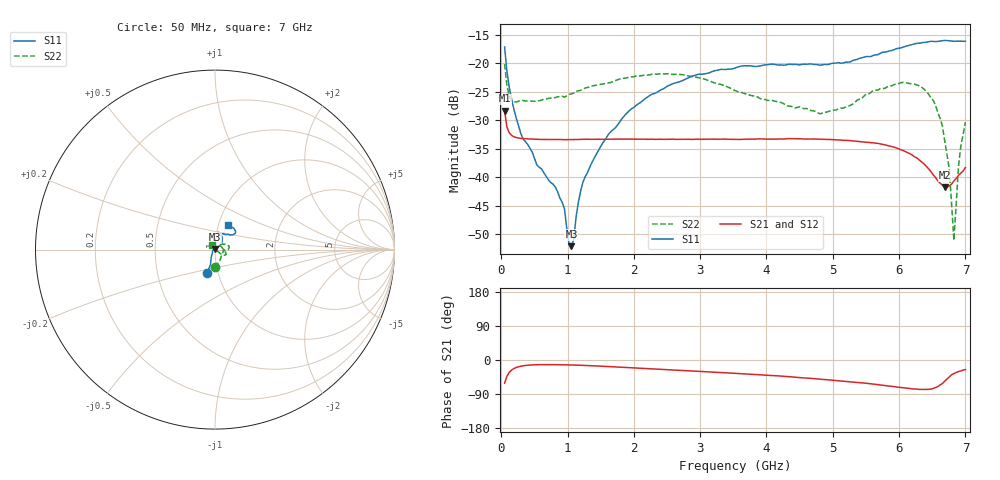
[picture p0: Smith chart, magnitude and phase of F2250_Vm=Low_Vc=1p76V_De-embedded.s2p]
! Integrated Device Technology
! Corporate Headquarters
! 6024 Silver Creek Valley Road
! San Jose, CA 95138  USA
! Phone:  1-408-284-8200
! Toll Free:  1-800-223-1366
! Webpage:  http://www.idt.com/
! Timing and RF Division
! 515 Groton Road, Suite 102
! Westford, MA 01886-6024
! Device:  F2250
! Description: Voltage Variable RF Attenuator
! Frequency:  50.0 -  6000.00 MHz
! Package:  3x3 mm Thin QFN Plastic Package: 16 pin
! Ports:  2 RF, 3 DC
!  Pin  1  = GND
!  Pin  2  = NC
!  Pin  3  = RF1  = Port 1
!  Pin  4  = NC
!  Pin  5  = GND
!  Pin  6  = GND
!  Pin  7  = GND
!  Pin  8  = GND
!  Pin  9  = NC
!  Pin 10  = RF2  = Port 2
!  Pin 11  = NC
!  Pin 12  = GND
!  Pin 13  = GND
!  Pin 14  = VCNTRL
!  Pin 15  = VDD
!  Pin 16  = VMODE
! Vcntrl:  1.760 Volts
! Vmode:  +0.000 Volts
! Vdd:  +3.30  Volts
! Current:  1.187 mA
! Data:  The device was measured on a the F2250 evaluation board which has
!  individual transmission lines to the RF pins.  Data was collected
!  using a calibrated network analyzer.  The evaluation board was
!  de-embedded using a TRL calibration technique.
!  The reference plane is the edge of the package pin.
! Misc:  SN 10
!  Action Tracker AT0258
! Date Measured:  2014-11-26
! Date:  2015-10-15  MJV
! Note:
!  Integrated Device Technology supplies this data as a sample of measured
!  data at the package pin for this product.  Your particular data for this
!  product may vary.
!  Data was taken at 25 degrees C.
!  Integrated Device Technology reserves the right to change this data at anytime.
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# GHz S dB R 50
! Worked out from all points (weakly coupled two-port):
!   201 points, 50 MHz to 7 GHz, reference 50 ohm
!   highest |S21| = -28.35 dB at 50 MHz (marker M1); lowest = -41.8 dB at 6.687 GHz (marker M2)
!   lowest |S11| = -52.1 dB at 1.058 GHz (marker M3), VSWR 1.00, Z = 49.9 + j0.226 ohm
!   |S11| at or under -10 dB: start of sweep to end of sweep
!   |S22| runs from -51.1 to -20.2 dB; largest |S21 - S12| = 6.9e-05
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0.05  -17.16 -108.2  -28.35 -60.9  -28.35 -60.9  -20.15 -90.9
0.1195  -24.20 -111.1  -32.20 -32.8  -32.21 -32.8  -25.74 -48.1
0.29325  -32.28 -126.4  -33.19 -16.4  -33.17 -16.4  -26.50 -19.9
0.5365  -37.85 -153.8  -33.36 -12.5  -33.37 -12.5  -26.66 -8.1
0.84925  -42.55 170.5  -33.40 -12.4  -33.40 -12.4  -25.88 -6.7
0.9535  -45.58 170.9  -33.42 -12.7  -33.41 -12.7  -25.96 -6.1
1.023  -51.85 140.3  -33.41 -13.0  -33.41 -13.0  -25.47 -4.9
1.05775  -52.11 114.0  -33.41 -13.1  -33.41 -13.1  -25.38 -4.4
1.2315  -40.88 40.9  -33.37 -14.1  -33.37 -14.1  -24.56 -5.6
1.6485  -32.05 40.7  -33.34 -17.4  -33.34 -17.4  -23.39 -0.3
2.37825  -24.88 46.8  -33.35 -24.1  -33.35 -24.1  -21.87 8.3
3.525  -20.84 72.2  -33.38 -35.0  -33.37 -35.0  -24.79 31.0
4.7065  -20.21 72.2  -33.30 -49.0  -33.30 -49.0  -28.34 38.2
5.15825  -19.96 57.7  -33.55 -55.9  -33.55 -55.9  -27.86 15.6
5.85325  -17.84 40.3  -34.52 -68.8  -34.52 -68.8  -24.03 -17.3
6.3745  -16.35 41.2  -37.66 -77.7  -37.67 -77.7  -24.52 -30.9
6.54825  -16.21 45.0  -40.04 -72.8  -40.09 -72.8  -27.34 -36.5
6.68725  -16.01 48.7  -41.79 -56.2  -41.76 -56.2  -33.58 -32.5
6.75675  -16.07 51.0  -41.56 -44.9  -41.51 -44.9  -38.54 -27.0
6.82625  -16.16 53.4  -40.67 -35.9  -40.64 -35.8  -51.10 62.6
6.89575  -16.12 57.0  -39.69 -30.5  -39.65 -30.5  -38.12 114.6
7  -16.15 63.1  -38.32 -25.2  -38.29 -25.2  -30.36 129.2
